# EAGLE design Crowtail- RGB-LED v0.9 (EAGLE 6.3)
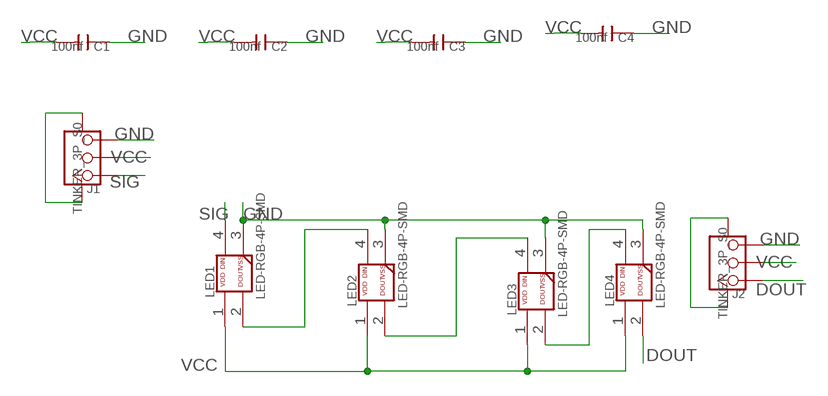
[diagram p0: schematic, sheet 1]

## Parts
C1  100nf  C-0603  [C0603]
C2  100nf  C-0603  [C0603]
C3  100nf  C-0603  [C0603]
C4  100nf  C-0603  [C0603]
J1  TINKER_3P_S0  [TINKER_3P_S0]
J2  TINKER_3P_S0  [TINKER_3P_S0]
LED1  LED-RGB-4P-SMD  [LED-RGB-4P-SMD]
LED2  LED-RGB-4P-SMD  [LED-RGB-4P-SMD]
LED3  LED-RGB-4P-SMD  [LED-RGB-4P-SMD]
LED4  LED-RGB-4P-SMD  [LED-RGB-4P-SMD]

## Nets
DOUT: J2.1 LED4.2
GND: C1.1 C2.1 C3.1 C4.1 J1.3 J1.SS1 J1.SS2 J2.3 J2.SS1 J2.SS2 LED1.3 LED2.3 LED3.3 LED4.3
N$11: LED1.2 LED2.4
N$12: LED2.2 LED3.4
N$13: LED3.2 LED4.4
SIG: J1.1 LED1.4
VCC: C1.2 C2.2 C3.2 C4.2 J1.2 J2.2 LED1.1 LED2.1 LED3.1 LED4.1

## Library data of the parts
C1-C4 = Discrete:C*: Ceramic Capacitors
J1 J2 = Connector:TINKER_3P_S0
LED1-LED4 = Discrete:LED-RGB-4P-SMD

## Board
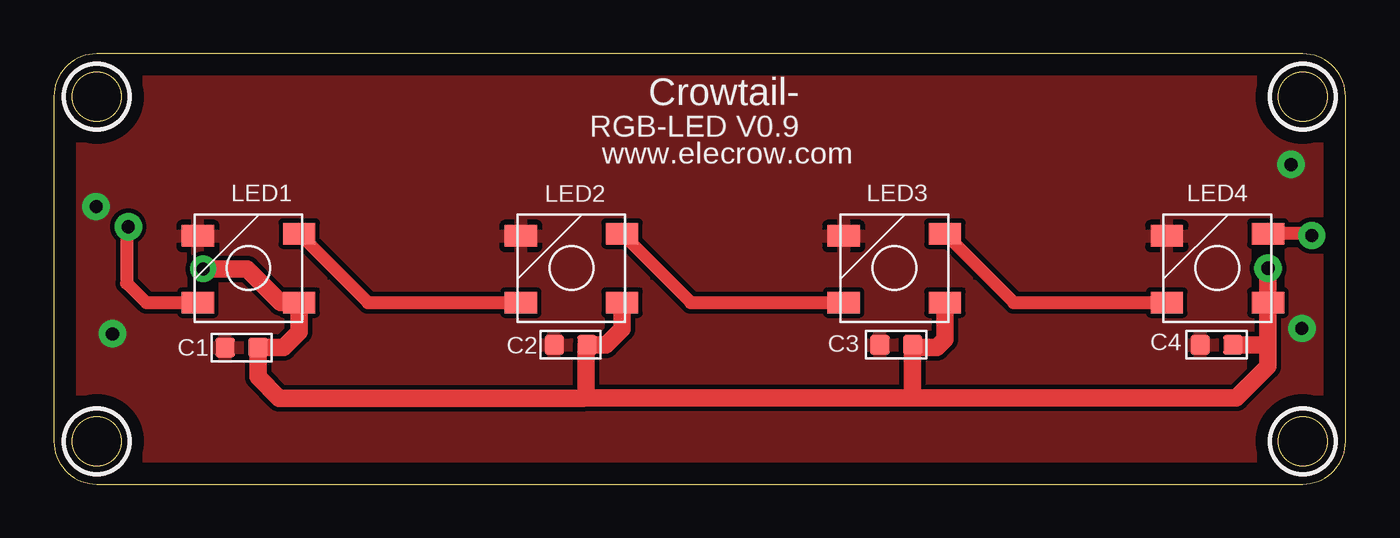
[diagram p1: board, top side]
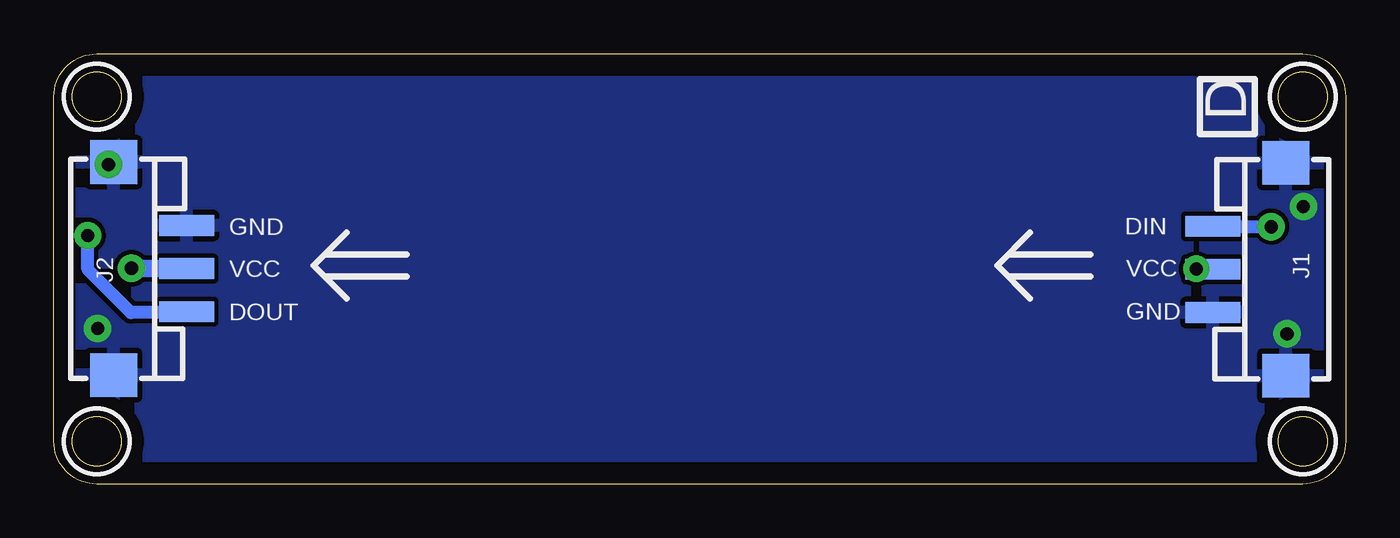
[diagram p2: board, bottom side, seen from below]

Size 60 x 20 mm. Coordinates in mm from the lower left corner, seen from the top.
Outline: 0,18 0,2 arc90 2,0 58,0 arc90 60,2 60,18 arc90 58,20 2,20 arc90 0,18
Outline: circle at 2,18 radius 1.14
Outline: circle at 2,2 radius 1.14
Outline: circle at 58,18 radius 1.14
Outline: circle at 58,2 radius 1.14
Copper layers (1*16): Top 0.035mm / dielectric 1.5mm / Bottom 0.035mm
Design rules "default *": minimum track width 10mil, minimum drill 24mil, track to track 8mil, track to pad 8mil, pad to pad 8mil, via to via 8mil, smd to smd 8mil, copper to edge 40mil, drill to drill 8mil, minimum pad ring 10mil, minimum via ring 8mil, stop-mask expansion 2mil, vias tented up to drill 100mil, thermal gap 10mil
tRestrict: area 0.5,16.5 to 3.5,19.5; area 0.5,0.5 to 3.5,3.5; area 56.5,16.5 to 59.5,19.5; area 56.5,0.5 to 59.5,3.5
bRestrict: area 0.5,16.5 to 3.5,19.5; area 0.5,0.5 to 3.5,3.5; area 56.5,16.5 to 59.5,19.5; area 56.5,0.5 to 59.5,3.5

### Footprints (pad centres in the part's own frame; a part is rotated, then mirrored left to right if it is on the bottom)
C0603 = smd 0.889 x 0.889: 1 -0.762,0; 2 0.762,0
TINKER_3P_S0 = smd 0.965 x 2.54: 1 -1.984,-3.175; 2 0.016,-3.175; 3 2.016,-3.175 | smd 2.032 x 2.184: SS1 -4.93,0.225; SS2 4.962,0.225
LED-RGB-4P-SMD = smd 1.5 x 1: 1 -2.39,1.56; 2 -2.39,-1.64; 3 2.31,-1.54; 4 2.31,1.56

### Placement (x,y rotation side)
C1  8.72,6.35 0 top
C2  24.01,6.48 0 top
C3  39.13,6.48 0 top
C4  54,6.48 0 top
J1  3,10 270 bottom
J2  57,10 90 bottom
LED1  9,10 180 top
LED2  24,10 180 top
LED3  39,10 180 top
LED4  54,10 180 top

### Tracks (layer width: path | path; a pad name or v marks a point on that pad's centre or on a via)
DOUT  (via drill 0.61 pad 1.27)
  Top 0.406: v58.42,11.56 58.34,11.64
  Top 0.61: 58.34,11.64 LED4.2
  Bottom 0.406: J2.1 53.87,7.98
  Bottom 0.61: 53.87,7.98 56.42,7.98 58.42,9.98 v58.42,11.56
GND  (via drill 0.61 pad 1.27)
  other vias: 1.96,12.9 2.72,6.99 57.97,7.24 57.46,14.86
  pour Top: -0.56,20.24 60.7,20.24 60.7,-0.28 -0.58,-0.28 -0.58,20.22
  pour Bottom: -0.66,20.5 60.61,20.5 60.61,-0.51 -0.69,-0.51 -0.69,20.52
N$11
  Top 0.61: LED1.2 14.59,8.44 LED2.4
N$12
  Top 0.61: LED2.2 29.59,8.44 LED3.4
N$13
  Top 0.61: LED3.2 44.59,8.44 LED4.4
SIG  (via drill 0.61 pad 1.27)
  Top 0.406: v3.46,11.96 3.54,11.89 3.38,11.73
  Top 0.61: 3.38,11.73 3.38,9.35 4.29,8.44 LED1.4
  Bottom 0.406: J1.1 6.15,11.96
  Bottom 0.61: 6.15,11.96 v3.46,11.96
VCC  (via drill 0.61 pad 1.22, 0.61 pad 1.27)
  Top 0.406: 40.06,6.35 C3.2 39.75,6.39 39.88,6.26 | C2.2 25.02,6.31 24.85,6.48 C2.2 | C1.2 9.53,6.31 | C2.2 | 24.72,4.15 24.57,4 24.55,3.99 | C2.2 24.74,6.45 24.72,6.45 | 39.86,4 39.88,4.03 | 39.88,6.43 39.89,6.43 | LED4.1
  Top 0.813: 56.39,6.48 56.39,5.46 54.93,4 39.86,4 24.57,4 | 56.39,6.48 LED4.1 | LED3.1 41.39,6.72 41.02,6.35 40.06,6.35 | LED2.1 26.39,7.21 25.65,6.48 C2.2 | C4.2 56.39,6.48 | 24.72,4.15 24.72,6.45 | 39.88,4.03 39.88,6.43 | 39.89,6.43 C3.2 | LED4.1 v56.39,10.03 | 24.55,3.99 10.47,3.99 9.48,4.97 C1.2 10.67,6.35 11.39,7.07 LED1.1 10.54,8.44 8.97,10.01 v6.94,10.01
  Bottom 0.406: v56.39,10.03 56.38,10.02 | J1.2 6.94,9.98 v6.94,10.01 | J2.2 53.84,10.03
  Bottom 0.61: 6.1,10.01 v6.94,10.01
  Bottom 0.813: 53.84,10.03 v56.39,10.03

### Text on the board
tPlace: Crowtail- | RGB-LED V0.9 | www.elecrow.com
bPlace: D | DIN | GND | VCC | VCC | GND | DOUT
